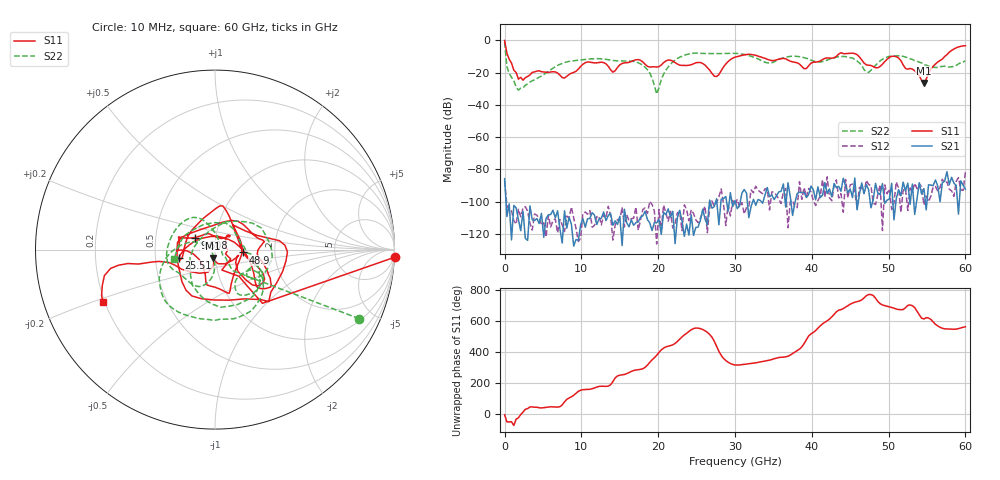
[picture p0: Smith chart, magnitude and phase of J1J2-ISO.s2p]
!Keysight Technologies,N5227A,US51270214,A.10.65.11
!Date: Thursday, October 15, 2020 08:10:11
!Correction: S11(Full 2 Port(1,2))
!S21(Full 2 Port(1,2))
!S12(Full 2 Port(1,2))
!S22(Full 2 Port(1,2))
!S2P File: Measurements: S11, S21, S12, S22:
# Hz S  dB  R 50
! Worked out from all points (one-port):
!   201 points, 10 MHz to 60 GHz, reference 50 ohm
!   lowest |S11| = -26.3 dB at 54.6 GHz (marker M1), VSWR 1.10, Z = 48.6 - j4.54 ohm
!   |S11| at or under -10 dB: 474.5 MHz to 30.31 GHz (29.83 GHz wide, 194 % of centre); 33.22 GHz to 43.15 GHz (9.936 GHz wide, 26 % of centre); 50.93 GHz to 57.29 GHz (6.361 GHz wide, 11.8 % of centre)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
!   S11 on the Smith chart (normalised r, x): 10 MHz: -1, -47; 9.608 GHz: 0.79, +0.11; 25.51 GHz: 0.66, -0.06; 48.9 GHz: 1.37, -0.04; 60 GHz: 0.19, -0.21
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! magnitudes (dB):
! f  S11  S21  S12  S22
! 10 MHz  0.0  -85.7  -87.2  -1.0
! 309.9 MHz  -8.0  -109.2  -102.0  -16.3
! 1.81 GHz  -24.0  -111.2  -104.7  -30.8
! 9.608 GHz  -17.7  -124.0  -124.8  -12.2
! 10.21 GHz  -14.7  -110.7  -107.0  -11.9
! 14.11 GHz  -19.7  -114.6  -123.9  -12.4
! 17.11 GHz  -12.0  -113.0  -103.4  -13.3
! 18.91 GHz  -16.5  -113.2  -99.8  -20.2
! 19.81 GHz  -16.5  -113.1  -126.3  -33.2
! 20.11 GHz  -16.2  -111.0  -104.9  -29.4
! 22.21 GHz  -13.7  -126.0  -113.6  -12.2
! 25.51 GHz  -13.7  -111.5  -110.2  -8.0
! 27.61 GHz  -22.4  -98.1  -100.7  -8.2
! 30 GHz  -10.3  -99.4  -101.8  -8.0
! 40.2 GHz  -13.4  -92.7  -99.3  -12.8
! 45.3 GHz  -7.9  -97.5  -89.1  -10.9
! 47.4 GHz  -15.4  -92.6  -89.3  -19.8
! 48.9 GHz  -16.1  -95.5  -89.5  -12.6
! 50.1 GHz  -10.5  -98.3  -92.2  -9.8
! 54.6 GHz  -26.3  -91.9  -102.1  -15.0
! 56.4 GHz  -13.3  -90.3  -93.5  -16.8
! 60 GHz  -3.2  -92.3  -81.8  -12.7
